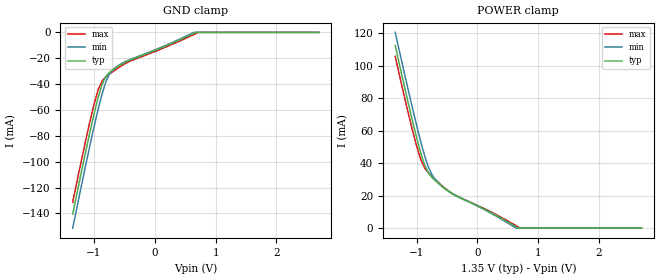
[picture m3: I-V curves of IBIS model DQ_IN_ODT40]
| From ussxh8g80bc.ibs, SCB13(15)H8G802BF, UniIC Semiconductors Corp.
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| MODEL DQ_IN_ODT40 (Data Input with 40ohm ODT, 800-2133Mbps)
[Model]   DQ_IN_ODT40
Model_type   Input
Vinl = 545.000mV
Vinh = 805.000mV
|   typ   min   max
|C_comp   0.965pF   0.916pF   1.023pF
C_comp_power_clamp   0.4825pF   0.4580pF   0.5115pF
C_comp_gnd_clamp   0.4825pF   0.4580pF   0.5115pF
| Note: C_comp changes when the ODT circuit is enabled.
[Model Spec]
| Input threshold voltage corners
Vinl   0.5450V   0.5115V   0.5825V
Vinh   0.8050V   0.7715V   0.8425V
| Dynamic Overshoot Parameters from DDR3L Specification
|D_overshoot_ampl_h   0.40   NA   NA
|D_overshoot_ampl_l   0.40   NA   NA
|D_overshoot_area_h   0.11n   NA   NA
|D_overshoot_area_l   0.11n   NA   NA
[Receiver Thresholds]
Vth   =  0.675V
Vth_min  =  0.6615V
Vth_max  =  0.6885V
Vinh_ac  =  0.130V
Vinh_dc  =  0.090V
Vinl_ac  = -0.130V
Vinl_dc  = -0.090V
Tslew_ac =  5.000ns |Not specified, so set to high value
Threshold_sensitivity = 0.50
Reference_supply Power_clamp_ref
[Voltage Range]   1.3500V   1.2830V   1.4250V
[POWER Clamp Reference]   1.3500V   1.2830V   1.4250V
| Junction Temperature (Ambient temp is 40C typ, 85C min, 0C max)
[Temperature Range]   45.0   90.0   0.0
[GND Clamp]
|   Voltage   I(typ)   I(min)   I(max)
-1.35V    -140.6mA   -151.4mA   -131.4mA
-1.075V   -78.79mA   -89.12mA   -70.46mA
-1.005V   -64.28mA   -74.23mA   -56.57mA
-935mV    -51mA      -60.09mA   -44.75mA
-875mV    -41.28mA   -49.01mA   -38.43mA
-800mV    -33.8mA    -37.59mA   -34.26mA
-745mV    -30.93mA   -32.17mA   -32.27mA
-640mV    -27.38mA   -26.98mA   -28.74mA
-400mV    -21.26mA   -20.92mA   -22.09mA
640mV     -769.1uA   -43.14uA   -1.721mA
720mV     0A         0A         0A
2.7V      0A         0A         0A
[POWER Clamp]
|   Voltage   I(typ)   I(min)   I(max)
-1.35V    112.5mA    120.7mA    105.9mA
-1.075V   67.44mA    75.32mA    61.57mA
-935mV    47.05mA    54.01mA    42.78mA
-875mV    39.82mA    45.82mA    37.75mA
-810mV    34.41mA    38.26mA    34.36mA
-750mV    31.45mA    33.22mA    32.04mA
-690mV    29.22mA    29.94mA    29.9mA
-550mV    24.74mA    24.87mA    25.23mA
-340mV    19.7mA     19.9mA     19.86mA
640mV     765.8uA    22.39uA    1.435mA
705mV     0A         0A         0A
2.7V      0A         0A         0A
